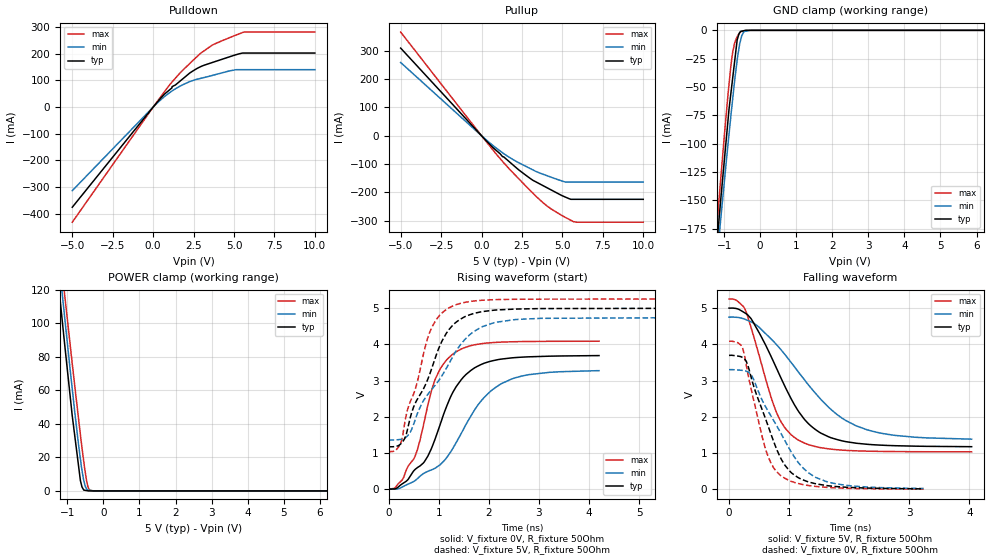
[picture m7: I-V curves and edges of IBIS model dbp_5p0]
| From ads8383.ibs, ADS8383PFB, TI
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|   dbp_5p0 Model
[Model]   dbp_5p0
Model_type   3-state
Polarity   Non-Inverting
Vmeas = 2.5
Vref = 2.5
Cref = 20pF
Rref = 50
|   typ   min   max
|   (nom PVT)   (fast PVT)   (slow PVT)
|C_comp from frequency sweep method (F=250KHz)
|C_comp   1.425e-11   1.192e-11   1.638e-11
|ON state : BUFFER OUTPUT TURNED HIGH
|C_comp   1.425e-11   1.192e-11   1.638e-11
|OFF state: BUFFER IN HIGH IMPEDANCE
|C_comp   2.117e-11   2.044e-11   2.185e-11
|C_comp from LC tank measurement(L=1nH)
|Resonant Frequency(Hz)   2.250e+09   2.370e+09   2.140e+09
C_comp   5.008e-12   4.514e-12   5.537e-12
|ON state : BUFFER OUTPUT TURNED HIGH
|Resonant Frequency(Hz)   2.250e+09   2.370e+09   2.140e+09
|C_comp   5.008e-12   4.514e-12   5.537e-12
|OFF state: BUFFER IN HIGH IMPEDANCE
|Resonant Frequency(Hz)   1.990e+09   1.990e+09   1.950e+09
|C_comp   6.403e-12   6.403e-12   6.668e-12
| Where nom  PVT is Nominal Process, 5V, 35C
|   Fast PVT is Strong Process,  5.25V, -30C
|   Slow PVT is Weak Process,   4.75V, 95C
[Voltage Range]   5   4.75   5.25
|Ambient Temperature   25   85   -40
|Junction Temperature
[Temperature Range]   35   95   -40
[Pullup Reference]   5   4.75   5.25
[Pulldown Reference]   0   0   0
[Power Clamp Reference]   5   4.75   5.25
[GND Clamp Reference]   0   0   0
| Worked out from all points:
|   slope of the pulldown table from 0 to 0.75 V, typ, clamps not added: 14.6 ohm
|   slope of the pullup table from 0 to 0.75 V, typ, clamps not added: 17.1 ohm
|   GND clamp passes 1 mA (typ) near -0.54 V on its own axis
|   POWER clamp passes 1 mA (typ) near -0.56 V on its own axis
|   falling waveform, V_fixture 5V, R_fixture 50Ohm: 20-80 % time 721ps typ, 1.06ns min, 484ps max; typ from 5 V to 1.18 V
|   rising waveform, V_fixture 0V, R_fixture 50Ohm: 20-80 % time 709ps typ, 961ps min, 518ps max; typ from 0 V to 3.69 V
|   rising waveform, V_fixture 5V, R_fixture 50Ohm: 20-80 % time 698ps typ, 924ps min, 514ps max; typ from 1.17 V to 5 V
|   falling waveform, V_fixture 0V, R_fixture 50Ohm: 20-80 % time 509ps typ, 680ps min, 367ps max; typ from 3.7 V to 0.013 V
[Pulldown]
|   Voltage   I(typ)   I(min)   I(max)
-5V       -375.6mA   -313.5mA   -431.7mA
475mV     33.93mA    27.68mA    39.14mA
1.165V    72.23mA    60.36mA    93.99mA
1.169V    76.62mA    60.49mA    94.22mA
1.596V    94.01mA    76.28mA    123.5mA
2.27V     128.1mA    95.69mA    163.8mA
2.94V     151.8mA    107.8mA    202.2mA
3.654V    167.1mA    118.6mA    232.3mA
4.731V    188.8mA    135.9mA    260.6mA
5.139V    196.7mA    140.3mA    270.5mA
5.602V    202.7mA    140.3mA    281.3mA
10V       202.7mA    140.3mA    281.3mA
[GND Clamp]
|   Voltage   I(typ)   I(min)   I(max)
-5V       -1.62A     -1.535A    -1.727A
-1.302V   -224.8mA   -236.7mA   -212.5mA
-1.123V   -160.2mA   -176.5mA   -142.4mA
-1.088V   -147.3mA   -164.5mA   -128.9mA
-865mV    -69.94mA   -92.04mA   -47.93mA
-803.3mV  -53.2mA    -72.54mA   -28.96mA
-714mV    -29.01mA   -46.29mA   -12.05mA
-640mV    -8.958mA   -26.9mA    -5.647mA
-545mV    -1.075mA   -8.977mA   -1.179mA
-451.2mV  -316.7uA   -1.174mA   -520.4uA
-270.7mV  -8.366uA   -5.228uA   -3.096uA
10V       0A         0A         0A
[Pullup]
|   Voltage   I(typ)   I(min)   I(max)
-5V       308.9mA    258.2mA    365.3mA
0V        0A         0A         0A
859.8mV   -49.26mA   -41.41mA   -61.08mA
1.305V    -73.91mA   -60.23mA   -90.79mA
1.596V    -85.62mA   -71.58mA   -109.5mA
2.715V    -138.2mA   -107.2mA   -176mA
3.165V    -156.7mA   -120.2mA   -201.9mA
4.058V    -183.6mA   -141mA     -247.9mA
5.178V    -216.1mA   -163.3mA   -287.7mA
5.525V    -224.2mA   -163.3mA   -298.1mA
5.691V    -224.2mA   -163.3mA   -303.1mA
10V       -224.2mA   -163.3mA   -304.8mA
[POWER Clamp]
|   Voltage   I(typ)   I(min)   I(max)
-5V       945.2mA    959.5mA    934.7mA
-1.306V   136.3mA    152.3mA    162.4mA
-1.085V   89.62mA    105.8mA    119.1mA
-865mV    44.89mA    61mA       76.07mA
-640mV    6.45mA     19.34mA    33.87mA
-595mV    2.375mA    12.33mA    25.91mA
-545mV    499.3uA    6.243mA    17.53mA
-503.5mV  341.2uA    2.7mA      11.22mA
-430.5mV  63.16uA    549.5uA    2.498mA
-383.2mV  3.536uA    382.9uA    431.5uA
-262.5mV  1.33uA     2.63uA     1.794uA
10V       0A         0A         0A
[Ramp]
R_load = 50
|   typ   min   max
dV/dt_r   2.2173/7.09353e-10   1.98008/9.68776e-10   2.45141/5.16037e-10
dV/dt_f   2.29865/7.23e-10   2.03568/1.07328e-09   2.52991/4.84423e-10
[Falling Waveform]
V_fixture = 5V
V_fixture_min = 4.75V
V_fixture_max = 5.25V
R_fixture = 50Ohm
|   Time   V(typ)   V(min)   V(max)
0s        5V         4.75V      5.25V
274ps     4.857V     4.687V     4.94V
400ps     4.618V     4.594V     4.278V
784ps     3.363V     4.005V     2.145V
956ps     2.752V     3.666V     1.645V
1.144ns   2.183V     3.262V     1.369V
1.528ns   1.551V     2.483V     1.149V
2.124ns   1.271V     1.747V     1.062V
2.77ns    1.203V     1.487V     1.042V
4.038ns   1.176V     1.384V     1.035V
[Rising Waveform]
V_fixture = 0V
V_fixture_min = 0V
V_fixture_max = 0V
R_fixture = 50Ohm
|   Time   V(typ)   V(min)   V(max)
0s        8.072nV    14.51nV    6.739nV
270ps     144.2mV    56.48mV    250mV
510ps     516.3mV    218.2mV    851.7mV
716ps     759.4mV    446mV      1.885V
942ps     1.435V     588.7mV    3.069V
1.286ns   2.681V     1.133V     3.733V
1.804ns   3.413V     2.361V     4.007V
2.254ns   3.593V     2.915V     4.061V
2.79ns    3.655V     3.161V     4.078V
4.2ns     3.689V     3.273V     4.085V
[Rising Waveform]
V_fixture = 5V
V_fixture_min = 4.75V
V_fixture_max = 5.25V
R_fixture = 50Ohm
|   Time   V(typ)   V(min)   V(max)
0s        1.169V     1.357V     1.033V
254ps     1.263V     1.376V     1.309V
374ps     1.623V     1.464V     2.167V
500ps     2.267V     1.788V     2.628V
860ps     3.327V     2.751V     4.457V
1.072ns   4.104V     3.145V     4.874V
1.324ns   4.583V     3.765V     5.082V
1.84ns    4.895V     4.466V     5.215V
2.52ns    4.973V     4.682V     5.244V
8.366ns   5V         4.75V      5.25V
[Falling Waveform]
V_fixture = 0V
V_fixture_min = 0V
V_fixture_max = 0V
R_fixture = 50Ohm
|   Time   V(typ)   V(min)   V(max)
0s        3.696V     3.301V     4.086V
228ps     3.636V     3.282V     3.889V
290ps     3.521V     3.26V      3.399V
376ps     3.042V     3.14V      2.708V
598ps     1.99V      2.311V     1.167V
702ps     1.505V     2.014V     712mV
860ps     861.6mV    1.556V     381.5mV
1.162ns   313.4mV    720.3mV    156.2mV
1.456ns   148.7mV    319mV      77.31mV
3.238ns   12.87mV    23.83mV    4.386mV
